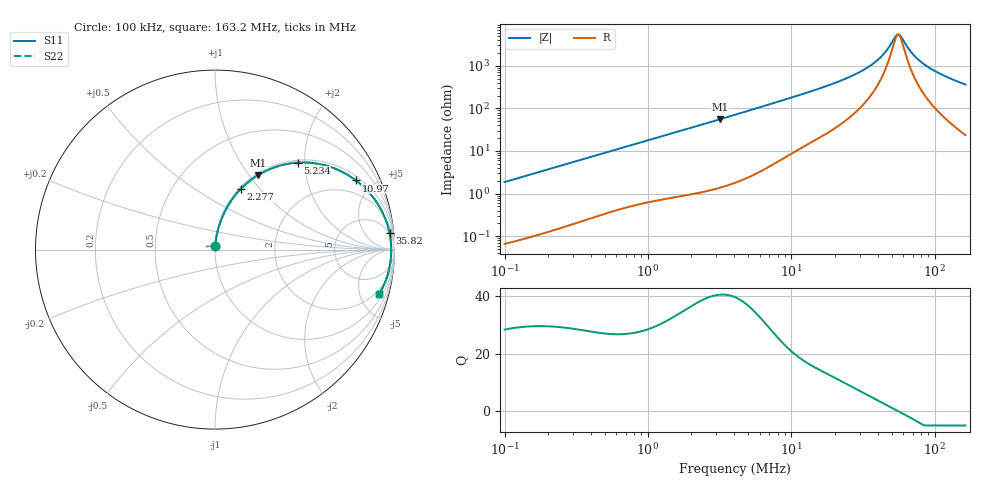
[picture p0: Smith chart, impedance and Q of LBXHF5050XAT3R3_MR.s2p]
! LBXHF5050XAT3R3_MR  S-PARAMETER MODEL  ( General Type )
! Model Generated by TAIYO YUDEN Corporation (http://www.ty-top.com)
! Version 1.0
! TAIYO YUDEN Control No. 200511NI43SB-FBB
! Copyright(c) 2020 TAIYO YUDEN CO.,LTD. All Rights Reserved.
! Product Description (link to TY-COMPAS)
! https://ds.yuden.co.jp/TYCOMPAS/or/detail?pn=LBXHF5050XAT3R3NMR&u=M
! Products Name : Inductors
! Characteristics :
!  Inductance : 3.3 uH , SRF(min) : 40 MHz , DC Resistance(max) : 0.037 Ohm
!  Rated Current : Saturation :4300 mA , Temp Rise : 2100 mA
!  Case Size : 5.0 x 5.0 / 0.197 x 0.197 [mm/inch] , Thickness : 3.1 / 0.122 [mm/inch]
!  (Conditions: Temperature = 25 degC , DC Bias Current/Voltage = 0A / 0V)
! External Node Assignments :
!  1  o---GGG---o  2
! GND o---------o GND
! Frequency Range : 0.1MHz  -  163.203978MHz  [ 402 STEP ]
# MHz S RI R 50
! Freq[MHz].  S11 Real  S11 Imag  S21 Real  S21 Imag  S12 Real  S12 Imag  S22 Real  S22 Imag
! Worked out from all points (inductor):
!   401 points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, 100 kHz to 163.2 MHz, reference 50 ohm
!   read as one part in series: L = 2.96 uH near 103.8 kHz
!   highest Q = 40.5 at 3.177 MHz (marker M1), where L = 2.79 uH
!   self-resonance near 54.81 MHz
!   S11 on the Smith chart (normalised r, x): 100 kHz: 1.00, +0.04; 2.277 MHz: 1.02, +0.80; 5.234 MHz: 1.05, +1.84; 10.97 MHz: 1.21, +3.96; 35.82 MHz: 5, +20; 163.2 MHz: 1.47, -7.27
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0.1  0.001 0.0186  0.999 -0.0186  0.999 -0.0186  0.001 0.0186
0.345249  0.00616 0.0625  0.9938 -0.0625  0.9938 -0.0625  0.00616 0.0625
0.671859  0.0186 0.1177  0.9814 -0.1177  0.9814 -0.1177  0.0186 0.1177
1.191969  0.0486 0.1989  0.9514 -0.1989  0.9514 -0.1989  0.0486 0.1989
2.277082  0.1437 0.3379  0.8563 -0.3379  0.8563 -0.3379  0.1437 0.3379
3.17652  0.2416 0.4159  0.7584 -0.4159  0.7584 -0.4159  0.2416 0.4159
4.115259  0.3462 0.4632  0.6538 -0.4632  0.6538 -0.4632  0.3462 0.4632
5.233726  0.4602 0.4846  0.5398 -0.4846  0.5398 -0.4846  0.4602 0.4846
7.301025  0.6225 0.4671  0.3775 -0.4671  0.3775 -0.4671  0.6225 0.4671
10.9669  0.785 0.3855  0.215 -0.3855  0.215 -0.3855  0.785 0.3855
13.94754  0.8534 0.3233  0.1466 -0.3233  0.1466 -0.3233  0.8534 0.3233
24.2914  0.9457 0.1796  0.0543 -0.1796  0.0543 -0.1796  0.9457 0.1796
30.32735  0.9639 0.1275  0.0361 -0.1275  0.0361 -0.1275  0.9639 0.1275
35.81962  0.9728 0.0907  0.0272 -0.0907  0.0272 -0.0907  0.9728 0.0907
42.30653  0.9785 0.0555  0.0215 -0.0555  0.0215 -0.0555  0.9785 0.0555
48.15376  0.981 0.0289  0.019 -0.0289  0.019 -0.0289  0.981 0.0289
53.80481  0.9819 0.00626  0.0181 -0.00626  0.0181 -0.00626  0.9819 0.00626
56.87437  0.982 -0.00501  0.018 0.00501  0.018 0.00501  0.982 -0.00501
69.70544  0.98 -0.0467  0.02 0.0467  0.02 0.0467  0.98 -0.0467
83.86581  0.9748 -0.0857  0.0252 0.0857  0.0252 0.0857  0.9748 -0.0857
112.7442  0.9581 -0.1527  0.0419 0.1527  0.0419 0.1527  0.9581 -0.1527
163.204  0.916 -0.2467  0.084 0.2467  0.084 0.2467  0.916 -0.2467
